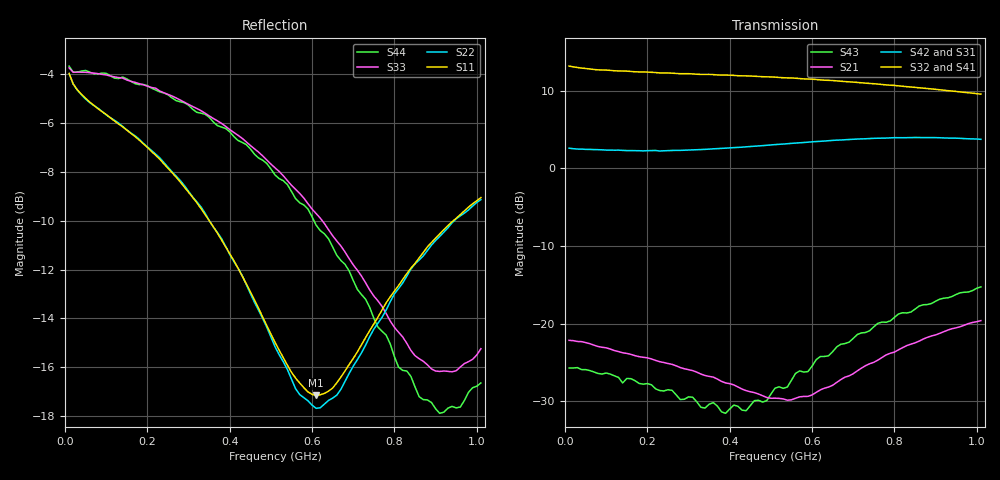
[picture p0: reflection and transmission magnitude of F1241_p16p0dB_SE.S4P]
! Integrated Device Technology
! Corporate Headquarters
! 6024 Silver Creek Valley Road
! San Jose, CA 95138  USA
! Phone:  1-408-284-8200
! Toll Free:  1-800-223-1366
! Webpage:  http://www.idt.com/
! Timing and RF Division
! 515 Groton Road, Suite 102
! Westford, MA 01886-6024
! Device:  F1241
! Description: Dual Intermediate Frequency Digital Variable Gain Amplifier
! Frequency:  10.0 -  500.00 MHz
! Package:  5x5 mm QFN Plastic Package: 32 pin
! Ports:  8 RF, 20 DC
!  Pin  1  = GA3  Pin 17  = RF OUT_B+
!  Pin  2  = GA4  Pin 18  = RF OUT_B-
!  Pin  3  = GA5  Pin 19  = STBY_B
!  Pin  4  = ISET_A  Pin 20  = Ground
!  Pin  5  = ISET_B  Pin 21  = Ground
!  Pin  6  = GB5  Pin 22  = STB_A
!  Pin  7  = GB4  Pin 23  = RF OUT_A-  = Port 4
!  Pin  8  = GB3  Pin 24  = RF OUT_A+  = Port 3
!  Pin  9  = GB2  Pin 25  = NO CONNECT
!  Pin 10  = GB1  Pin 26  = NO CONNECT
!  Pin 11  = RF IN_B+  Pin 27  = VCC
!  Pin 12  = RF IN_B-  Pin 28  = Ground
!  Pin 13  = Ground  Pin 29  = RF IN_A-  = Port 2
!  Pin 14  = VCC  Pin 30  = RF IN_A+  = Port 1
!  Pin 15  = NO CONNECT  Pin 31  = GA1
!  Pin 16  = NO CONNECT  Pin 32  = GA2
! State:  4
! Gain State:  16.0 dB
! Voltages:  Vcc = +5.00 Volts  Icc approximately 160.0 mA or 80 mA per channel.
! Data:  The device was measured on a custom evaluation board which has
!  individual transmission lines to the RF pins.  Data was collected
!  using a calibrated network analyzer.  The evaluation board was
!  de-embedded using a port reference technique.
!  The reference plane is the edge of the package pin.
!  Only Channel A was measured.
!  This data is in single-ended operation.  If your needs are balanced
!  or differential S-parameters then this file needs to be used a
!  linear simulator.
! Misc:  Lot Code  160028MY
!  Action Tracker AT004
! Date Measured:  2014-08-14
! Date:  2014-08-28  MJV
! Note:
!  Integrated Device Technology supplies this data as a sample of measured
!  data at the package pin for this product.  Your particular data for this
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# Hz S dB R 50
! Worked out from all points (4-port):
!   101 points, 10 MHz to 1.01 GHz, reference 50 ohm
!   strongest paths, dB at 10 MHz, 260 MHz, 510 MHz, 760 MHz, 1.01 GHz:
!     S32: 13.2, 12.3, 11.8, 10.9, 9.6
!     S41: 13.2, 12.2, 11.6, 10.7, 9.3
!     S42: 2.6, 2.3, 3.1, 3.9, 3.8
!     S31: 2.6, 2.2, 2.8, 3.6, 3.5
!     S21: -22.2, -25.2, -29.6, -24.7, -19.6
!     S43: -25.7, -28.6, -28.3, -20.0, -15.3
!   lowest |S11| = -17.2 dB at 610 MHz (marker M1), VSWR 1.32, Z = 39.8 - j7.12 ohm
!   |S11| at or under -10 dB: 350.4 MHz to 942.9 MHz (592.5 MHz wide, 91.6 % of centre)
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1e7  -3.96 -11.4  -22.15 7.4  -48.69 38.0  -22.89 6.8
     -22.15 7.3  -3.97 -11.3  -22.91 6.6  -48.80 38.3
     2.61 3.4  13.19 -175.3  -3.73 -8.1  -25.80 18.3
     13.21 -175.2  2.62 3.5  -25.72 17.3  -3.66 -8.2
5e7  -4.98 -13.6  -22.50 -11.0  -43.78 53.6  -23.23 -2.9
     -22.44 -11.1  -5.01 -13.2  -23.17 -2.8  -43.95 55.0
     2.48 -4.8  12.89 172.4  -3.91 -5.5  -26.19 -7.3
     12.89 172.0  2.47 -4.7  -25.92 -6.0  -3.84 -5.5
2.5e8  -7.85 -40.0  -25.18 -44.3  -31.82 54.7  -23.35 -8.2
       -25.14 -46.9  -7.81 -38.1  -23.31 -8.6  -31.81 54.1
       2.19 -21.7  12.31 146.1  -4.82 -20.6  -27.84 -56.8
       12.25 145.4  2.30 -21.4  -28.52 -51.4  -4.84 -19.8
4.4e8  -12.58 -73.8  -28.74 -89.0  -27.40 37.3  -22.57 -16.3
       -28.64 -95.4  -12.60 -70.8  -22.45 -16.2  -27.33 36.4
       2.53 -36.1  11.94 122.7  -6.76 -36.3  -27.31 -123.4
       11.82 121.6  2.79 -36.8  -31.22 -130.6  -6.88 -34.5
6.1e8  -17.17 -140.7  -30.37 -169.8  -25.16 20.2  -21.96 -27.8
       -28.86 -173.2  -17.69 -138.6  -21.73 -27.8  -25.06 18.4
       3.18 -52.0  11.47 101.2  -9.71 -54.1  -23.54 178.3
       11.30 100.3  3.47 -53.9  -24.64 160.9  -10.19 -50.8
8e8  -12.88 151.4  -24.73 126.8  -23.82 1.8  -21.87 -43.3
     -23.67 123.6  -13.00 151.6  -21.51 -43.4  -23.71 -0.6
     3.72 -74.3  10.70 77.7  -14.37 -87.1  -18.74 131.8
     10.48 76.8  3.97 -77.1  -19.20 118.0  -15.57 -84.0
1.01e9  -9.05 126.6  -20.22 89.0  -23.12 -15.9  -22.59 -59.7
        -19.61 87.1  -9.14 127.3  -22.02 -59.9  -22.94 -19.3
        3.54 -102.3  9.58 52.7  -15.25 -154.0  -15.35 94.2
        9.33 51.9  3.76 -105.7  -15.26 81.8  -16.65 -158.9
